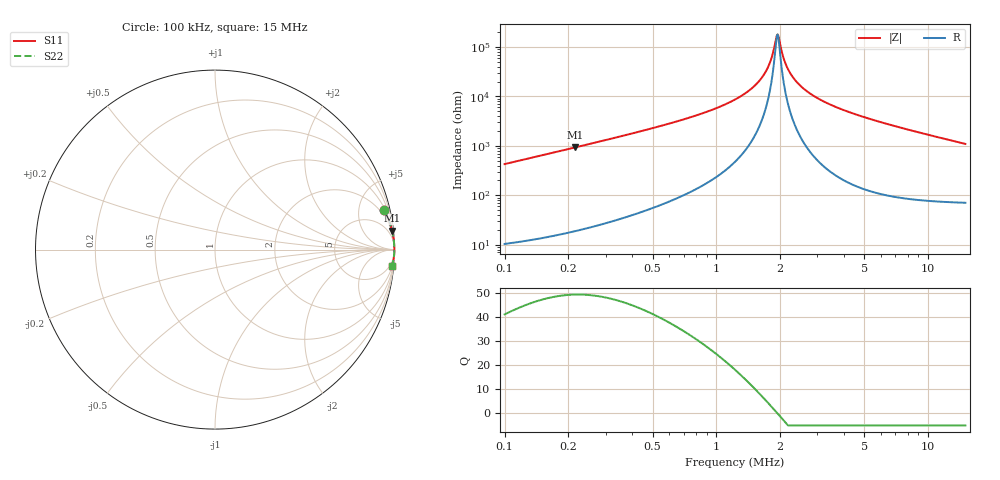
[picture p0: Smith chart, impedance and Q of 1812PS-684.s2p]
# MHz S MA R 50
!Freq  MagS11  AngS11  MagS21  AngS21  MagS12  AngS12  MagS22  AngS22
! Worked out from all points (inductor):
!   801 points, 100 kHz to 15 MHz, reference 50 ohm
!   read as one part in series: L = 680 uH near 102.5 kHz
!   highest Q = 49.4 at 216.1 kHz (marker M1), where L = 688 uH
!   self-resonance near 1.935 MHz
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0.1  0.9686 13.1  0.2261 -75.5  0.2261 -75.5  0.9686 13.1
0.2160598  0.9922 6.1  0.1062 -82.7  0.1062 -82.7  0.9922 6.1
0.3434492  0.9964 3.8  0.06579 -85.0  0.06579 -85.0  0.9964 3.8
0.516024  0.9981 2.4  0.04209 -86.2  0.04209 -86.2  0.9981 2.4
1.279636  0.9993 0.6  0.01038 -86.0  0.01038 -86.0  0.9993 0.6
1.563616  0.9994 0.3  0.00532 -83.4  0.00532 -83.4  0.9994 0.3
1.761214  0.9994 0.1  0.002454 -76.6  0.002454 -76.6  0.9994 0.1
1.82866  0.9994 0.1  0.001584 -69.2  0.001584 -69.2  0.9994 0.1
1.910617  0.9994 0.0  0.0007011 -37.4  0.0007011 -37.4  0.9994 0.0
1.934701  0.9994 0.0  0.0005699 -12.6  0.0005699 -12.6  0.9994 0.0
1.971398  0.9994 -0.0  0.0006446 30.5  0.0006446 30.5  0.9994 -0.0
2.085717  0.9994 -0.1  0.001773 71.7  0.001773 71.7  0.9994 -0.1
2.206665  0.9994 -0.2  0.003097 79.5  0.003097 79.5  0.9994 -0.2
2.378908  0.9994 -0.3  0.004912 83.2  0.004912 83.2  0.9994 -0.3
2.596924  0.9994 -0.4  0.007076 85.0  0.007076 85.0  0.9994 -0.4
2.980587  0.9994 -0.6  0.0106 86.2  0.0106 86.2  0.9994 -0.6
3.507719  0.9992 -0.9  0.01503 86.7  0.01503 86.7  0.9992 -0.9
5.075882  0.9987 -1.5  0.02677 86.5  0.02677 86.5  0.9987 -1.5
7.578772  0.9974 -2.5  0.04369 85.3  0.04369 85.3  0.9974 -2.5
10.04625  0.9955 -3.4  0.05953 83.9  0.05953 83.9  0.9955 -3.4
12.58717  0.993 -4.3  0.07542 82.5  0.07542 82.5  0.993 -4.3
15  0.9901 -5.2  0.09021 81.1  0.09021 81.1  0.9901 -5.2
